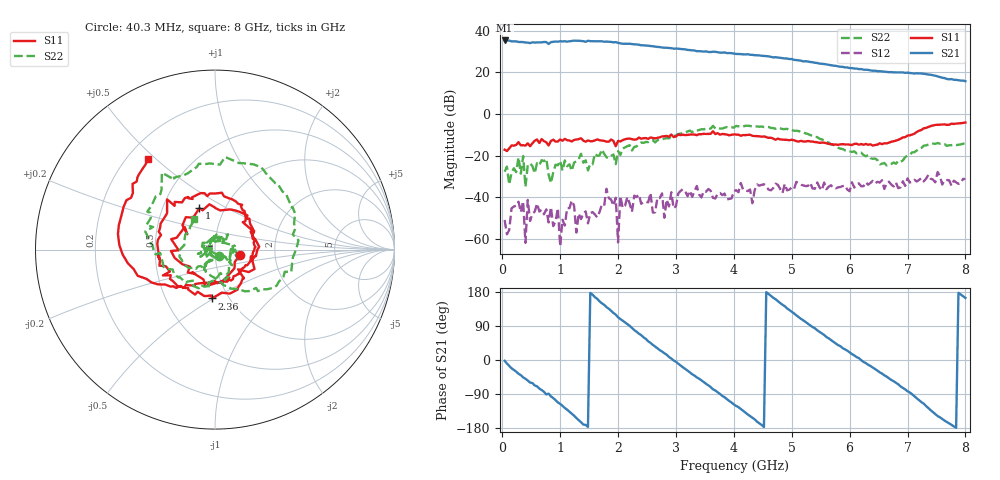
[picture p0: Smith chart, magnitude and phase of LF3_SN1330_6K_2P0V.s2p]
! VC=2.0V I=13.7mA
# HZ S DB R 50.00
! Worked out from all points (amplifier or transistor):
!   200 points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, 40.3 MHz to 8 GHz, reference 50 ohm
!   highest |S21| = 35.3 dB at 40.3 MHz (marker M1)
!   |S21| within 3 dB of that: start of sweep to 2.653 GHz
!   unconditionally stable (mu >= 1): start of sweep to 1.799 GHz; 1.803 GHz to 3.63 GHz; 4.529 GHz to end of sweep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
!   at 1.36 GHz: K = 2.78, MAG = 35.4 dB, |S12| = -50.4 dB
!   at 4.04 GHz: K = 1.08, MAG = 31.0 dB, |S12| = -36.5 dB
!   at 8 GHz: K = 1.82, MAG = 18.2 dB, |S12| = -31.2 dB
!   S11 on the Smith chart (normalised r, x): 40.3 MHz: 1.31, -0.08; 1 GHz: 0.76, +0.37; 2.36 GHz: 0.84, -0.49; 8 GHz: 0.28, +0.47
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4.02985e7  -17.07 -12.9  35.28 -2.1  -50.76 -142.0  -27.62 -55.2
1.60294e8  -15.08 -72.8  34.85 -21.9  -45.17 164.3  -28.08 -136.7
3.602865e8  -14.93 -135.2  34.50 -45.9  -41.89 131.8  -20.11 -166.0
7.20273e8  -13.01 162.9  34.55 -84.0  -48.06 53.0  -22.58 167.5
8.0027e8  -15.07 151.0  33.59 -88.8  -51.96 -112.9  -28.97 130.2
1.000262e9  -12.16 110.7  34.91 -115.9  -63.35 -109.1  -22.43 91.9
1.240254e9  -12.42 69.2  35.20 -146.9  -43.88 22.4  -23.29 48.5
1.400248e9  -12.75 43.2  34.94 -170.3  -47.71 96.4  -23.34 35.2
1.640238e9  -12.16 3.7  34.90 161.3  -49.53 76.5  -20.03 11.0
1.960226e9  -15.44 -40.6  34.49 119.6  -40.13 61.9  -24.00 -35.8
2.360212e9  -11.30 -93.4  33.23 69.4  -38.62 -76.8  -14.48 -101.7
2.720198e9  -11.15 -131.0  32.12 26.1  -40.27 -66.6  -12.16 -131.1
3.040186e9  -9.83 -163.9  31.31 -9.8  -38.09 -90.4  -9.58 -175.4
3.520168e9  -9.55 148.3  30.03 -62.9  -37.23 -138.6  -7.06 138.1
4.040148e9  -9.86 102.1  28.81 -121.3  -36.50 -169.9  -5.70 83.7
4.600128e9  -11.42 54.9  27.66 174.3  -36.22 132.3  -6.21 24.1
5.000112e9  -12.32 25.8  26.39 127.4  -35.18 88.3  -7.74 -21.7
5.360099e9  -13.21 -1.5  24.84 87.0  -35.69 88.9  -10.36 -49.3
5.960076e9  -14.56 -46.9  22.36 24.7  -36.22 20.3  -17.49 -113.1
6.68005e9  -13.72 -114.3  20.08 -48.4  -32.43 -36.9  -24.14 -104.6
7.400022e9  -5.77 -176.8  18.85 -132.4  -30.98 -85.3  -14.33 -154.3
8e9  -4.06 126.5  15.77 163.8  -31.19 -172.8  -13.72 124.6
